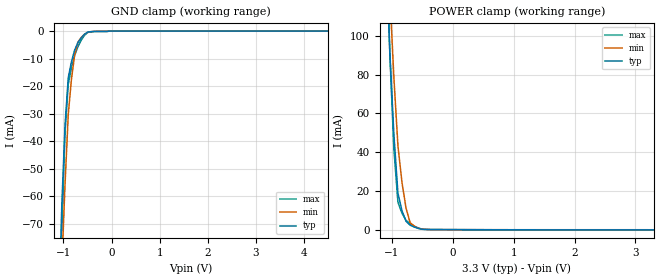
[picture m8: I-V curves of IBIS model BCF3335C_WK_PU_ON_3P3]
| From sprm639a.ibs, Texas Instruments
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|BCF3335C_WK_PD_ON_3P3; WEAK_PULLDOWN_ON
|   Model Cell BCF3335C_WK_PU_ON_3P3
|BCF3335C_WK_PU_ON_3P3
[Model]   BCF3335C_WK_PU_ON_3P3
Model_type   Input
Polarity   Non-Inverting
Vinl =  0.8
Vinh =  2
C_comp   1.21278p   1.078036p   1.350148p
[Model Spec]
Vinl   0.8   0.8   0.8
Vinh   2   2   2
[Temperature Range]   25   155   -40
[Voltage Range]   3.3   2.97   3.63
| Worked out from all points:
|   GND clamp passes 1 mA (typ) near -0.55 V on its own axis
|   POWER clamp passes 1 mA (typ) near -0.60 V on its own axis
| Nom Voltages:
|   VDD=1.2, VDDS=3.3, VSS=0
| Min Voltages:
|   VDD=1.08, VDDS=2.97, VSS=0
| Max Voltages:
|   VDD=1.32, VDDS=3.63, VSS=0
[POWER_clamp]
|   voltage   I(typ)   I(min)   I(max)
-3.3V     2.319A     2.596A     3.052A
-1.1V     147.6mA    172.2mA    162.5mA
-1.033V   92.43mA    121.8mA    91.34mA
-966.7mV  49.53mA    78.89mA    41.89mA
-900mV    18.88mA    43.52mA    14.19mA
-833.3mV  9.821mA    24.39mA    8.479mA
-766.7mV  4.304mA    11.1mA     4.78mA
-700mV    2.33mA     3.649mA    3.088mA
-566.7mV  645.6uA    749.7uA    841uA
-500mV    187.9uA    260.4uA    219.7uA
-366.7mV  40.03uA    41.85uA    52.54uA
3.3V      -108.8uA   -62.59uA   -174uA
[GND_clamp]
|   voltage   I(typ)   I(min)   I(max)
-3.3V     -1.89A     -1.587A    -3.158A
-1.1V     -103.3mA   -119.1mA   -124.2mA
-1.033V   -62.96mA   -85.24mA   -71.87mA
-966.7mV  -34.2mA    -55.64mA   -36.91mA
-900mV    -16.96mA   -30.35mA   -19.34mA
-833.3mV  -11.12mA   -17.43mA   -13.37mA
-766.7mV  -6.869mA   -8.657mA   -8.827mA
-700mV    -4.212mA   -4.029mA   -5.715mA
-566.7mV  -1.238mA   -1.201mA   -1.653mA
-500mV    -399.1uA   -475uA     -506.7uA
-33.33mV  0A         0A         0A
6.6V      0A         0A         0A
